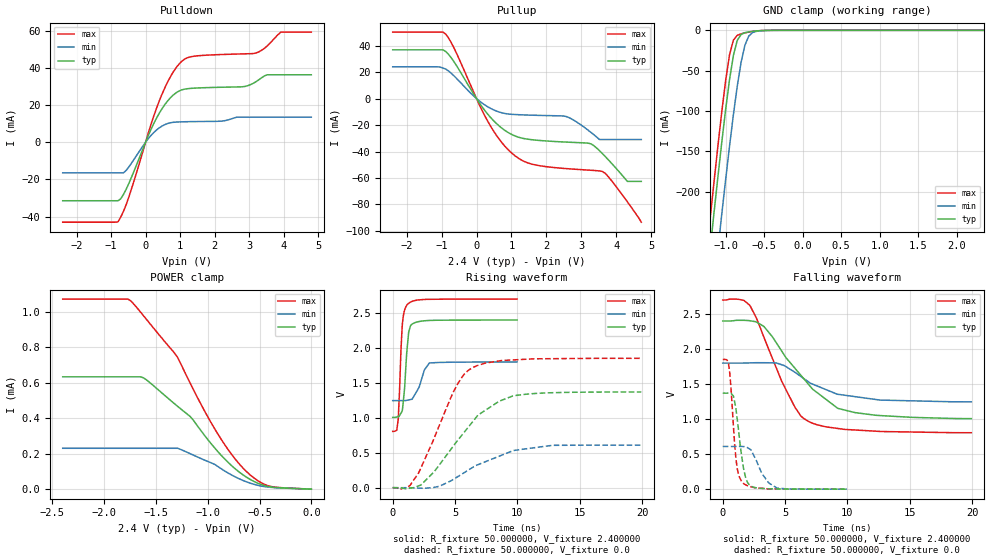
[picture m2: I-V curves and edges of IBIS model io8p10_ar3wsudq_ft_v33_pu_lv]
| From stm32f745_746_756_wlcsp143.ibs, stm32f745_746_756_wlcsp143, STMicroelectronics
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|   Model io8p10_ar3wsudq_ft_v33_pu_lv
[Model]  io8p10_ar3wsudq_ft_v33_pu_lv
Model_type I/O
Polarity   Non-Inverting
Enable   Active-Low
Vinl =   0.720000V
Vinh =   1.680000V
Vmeas =  1.200000V
Cref =   40.000000pF
Rref =   100.000000M
Vref =   0.0V
C_comp   3.739800pF   3.690400pF   3.817400pF
[Temperature Range]   25.000000   0.125000k   -40.000000
[Pullup Reference]   2.400000V   1.800000V   2.700000V
[Pulldown Reference]   0.0V   0.0V   0.0V
[POWER Clamp Reference]   2.400000V   1.800000V   2.700000V
[GND Clamp Reference]   0.0V   0.0V   0.0V
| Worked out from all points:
|   slope of the pulldown table from 0 to 0.36 V, typ, clamps not added: 25 ohm
|   slope of the pullup table from 0 to 0.36 V, typ, clamps not added: 27.7 ohm
|   GND clamp passes 1 mA (typ) near -0.62 V on its own axis
|   rising waveform, R_fixture 50.000000, V_fixture 2.400000: 20-80 % time 349ps typ, 701ps min, 271ps max; typ from 1.01 V to 2.4 V
|   rising waveform, R_fixture 50.000000, V_fixture 0.0: 20-80 % time 3.81ns typ, 4.17ns min, 2.72ns max; typ from 0.001 V to 1.37 V
|   falling waveform, R_fixture 50.000000, V_fixture 2.400000: 20-80 % time 4.08ns typ, 3.55ns min, 2.78ns max; typ from 2.4 V to 1.01 V
|   falling waveform, R_fixture 50.000000, V_fixture 0.0: 20-80 % time 601ps typ, 1.09ns min, 463ps max; typ from 1.37 V to 0.001 V
[Pulldown]
|Voltage   I(typ)   I(min)   I(max)
-2.4V     -31.47mA   -16.45mA   -43.01mA
-800mV    -31.47mA   -16.45mA   -42.85mA
-480mV    -21.98mA   -13.17mA   -29.21mA
80mV      3.63mA     1.966mA    5.014mA
480mV     18.16mA    8.738mA    26.02mA
800mV     25.38mA    10.72mA    37.77mA
1.12V     28.53mA    11.02mA    44.6mA
2.8V      29.84mA    13.47mA    47.53mA
3.2V      32.6mA     13.47mA    48.03mA
3.52V     36.3mA     13.47mA    51.75mA
3.92V     36.3mA     13.47mA    59.27mA
4.8V      36.3mA     13.47mA    59.27mA
[Pullup]
|Voltage   I(typ)   I(min)   I(max)
-2.4V     36.82mA    24mA       50.21mA
-960mV    36.82mA    23.01mA    50.21mA
-640mV    27.62mA    17.03mA    37.94mA
320mV     -11.75mA   -6.207mA   -17.08mA
640mV     -20.52mA   -10.1mA    -30.35mA
960mV     -26.47mA   -11.82mA   -40.02mA
1.52V     -30.88mA   -12.51mA   -49.05mA
2.56V     -32.88mA   -13.52mA   -52.9mA
3.28V     -34.25mA   -25.62mA   -54.17mA
3.6V      -41.44mA   -30.96mA   -55.02mA
4.32V     -62.57mA   -30.96mA   -77.98mA
4.72V     -62.57mA   -30.96mA   -93.4mA
[GND_clamp]
|Voltage   I(typ)   I(min)   I(max)
-2.4V     -1.437A    -1.518A    -1.411A
-1.25V    -315.9mA   -407.2mA   -278.2mA
-1.2V     -270.1mA   -361.3mA   -232.1mA
-1.15V    -225mA     -316mA     -186.8mA
-1.1V     -180.9mA   -271.3mA   -142.7mA
-1.05V    -138.2mA   -227.5mA   -100.5mA
-950mV    -61.14mA   -143.6mA   -30.43mA
-900mV    -31.23mA   -104.7mA   -12.14mA
-850mV    -12.49mA   -69.4mA    -6.221mA
-750mV    -2.898mA   -18.35mA   -3.18mA
-600mV    -750.2uA   -1.218mA   -738.3uA
2.35V     0A         0A         0A
[POWER_clamp]
|Voltage   I(typ)   I(min)   I(max)
-2.4V     634.4uA    230.9uA    1.073mA
-1.77V    634.4uA    230.9uA    1.073mA
-1.74V    634.4uA    230.9uA    1.062mA
-1.62V    628.7uA    230.9uA    979.3uA
-1.29V    467.4uA    230.9uA    743.1uA
-1.17V    410.9uA    200.6uA    599.2uA
-930mV    230.8uA    139uA      338.2uA
-780mV    138.4uA    83.46uA    204.6uA
-660mV    81.05uA    49.28uA    119.5uA
-540mV    39.7uA     25.07uA    57.27uA
-420mV    15.59uA    11.9uA     19.92uA
0V        0A         0A         0A
[Ramp]
| variable   typ   min   max
dV/dt_r  0.82207/3.80902n   0.36580/4.16677n   1.11359/2.72660n
dV/dt_f  0.83208/4.06970n   0.33384/3.68425n   1.13587/2.77844n
R_load = 50.000000
[Rising Waveform]
R_fixture= 50.000000
V_fixture= 2.400000
V_fixture_min= 1.800000
V_fixture_max= 2.700000
|time   V(typ)   V(min)   V(max)
0s        1.007V     1.247V     806mV
320.3ps   1.011V     1.247V     822.6mV
440.4ps   1.016V     1.247V     973.3mV
660.7ps   1.067V     1.247V     1.965V
760.8ps   1.097V     1.247V     2.311V
961ps     1.444V     1.247V     2.545V
1.201ns   2.076V     1.254V     2.627V
1.441ns   2.322V     1.263V     2.658V
2.943ns   2.393V     1.785V     2.696V
9.97ns    2.4V       1.8V       2.7V
[Rising Waveform]
R_fixture= 50.000000
V_fixture= 0.0
V_fixture_min= 0.0
V_fixture_max= 0.0
|time   V(typ)   V(min)   V(max)
0s        957.5uV    875.2uV    1.139mV
1.361ns   -6.151mV   380.2uV    28.19mV
2.082ns   26.77mV    -5.299mV   213.7mV
3.323ns   228mV      5.782mV    710.2mV
4.885ns   601.7mV    121.9mV    1.378V
5.646ns   774.5mV    206.4mV    1.605V
6.446ns   952.5mV    295.4mV    1.722V
9.65ns    1.315V     530.6mV    1.829V
12.81ns   1.36V      607.2mV    1.847V
19.94ns   1.371V     610.3mV    1.852V
[Falling Waveform]
R_fixture= 50.000000
V_fixture= 2.400000
V_fixture_min= 1.800000
V_fixture_max= 2.700000
|time   V(typ)   V(min)   V(max)
0s        2.4V       1.8V       2.7V
1.682ns   2.41V      1.8V       2.695V
2.202ns   2.403V     1.802V     2.616V
3.323ns   2.318V     1.805V     2.161V
4.725ns   1.973V     1.777V     1.543V
5.806ns   1.723V     1.667V     1.167V
6.887ns   1.496V     1.531V     967.1mV
9.209ns   1.157V     1.355V     867.3mV
10.61ns   1.093V     1.321V     845.1mV
19.94ns   1.007V     1.247V     806mV
[Falling Waveform]
R_fixture= 50.000000
V_fixture= 0.0
V_fixture_min= 0.0
V_fixture_max= 0.0
|time   V(typ)   V(min)   V(max)
0s        1.371V     610.3mV    1.852V
460.5ps   1.371V     610.2mV    1.796V
660.7ps   1.368V     610.1mV    1.449V
860.9ps   1.329V     610mV      893.3mV
1.181ns   976.2mV    609.8mV    282mV
1.622ns   352mV      609.2mV    90.77mV
2.242ns   47.91mV    565mV      36.33mV
3.143ns   11.9mV     224.3mV    12.89mV
4.364ns   4.599mV    15.72mV    4.396mV
9.97ns    957.5uV    875.2uV    1.139mV
